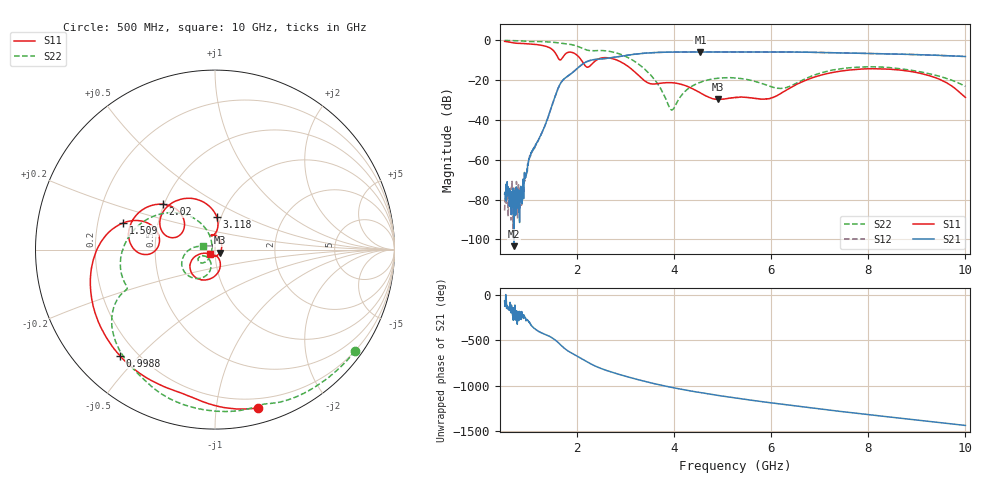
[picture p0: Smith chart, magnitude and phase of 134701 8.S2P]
!  2-Port S-parameters saved by WinCal
! VAR MeasName=S-Parameters (CALIBRATED_DATA) read from VNA (N5242A)
! VAR MeasDate=2013-7-3 16:23:51
! VAR NAME=134701 8
! VAR FILENAME=134701 8.S2P
! VAR DATE=2013-7-3 16:23:51
! VAR PHYS_PORTS=1,2
# Hz S MA R 50
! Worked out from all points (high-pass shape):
!   1601 points, 500 MHz to 10 GHz, reference 50 ohm
!   highest |S21| = -6.07 dB at 4.537 GHz (marker M1); lowest = -103.3 dB at 695.9 MHz (marker M2)
!   |S21| within 3 dB of the highest: 2.671 GHz to end of sweep
!   lowest |S11| = -29.8 dB at 4.9 GHz (marker M3), VSWR 1.07, Z = 52.8 - j1.8 ohm
!   |S11| at or under -10 dB: 1.633 GHz to 1.658 GHz (24.43 MHz wide, 1.49 % of centre); 2.077 GHz to 2.404 GHz (327.1 MHz wide, 14.6 % of centre); 2.799 GHz to end of sweep
!   |S22| runs from -35.2 to -0.3 dB; largest |S21 - S12| = 0.0018
!   S11 on the Smith chart (normalised r, x): 500 MHz: 0.12, -1.30; 998.8 MHz: 0.14, -0.44; 1.509 GHz: 0.31, +0.13; 2.02 GHz: 0.49, +0.29; 3.118 GHz: 0.95, +0.36; 10 GHz: 0.95, -0.05
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5e8  0.9137 -74.9  0.0001384 -68.9  5.323e-05 148.5  0.9632 -35.9
6.959375e8  0.8312 -99.3  6.8e-06 -173.9  0.0001253 135.1  0.9513 -49.8
8.503125e8  0.8112 -115.3  0.0001051 175.3  7.243e-05 95.9  0.9374 -60.9
9.9875e8  0.7937 -132.0  0.001044 65.2  0.0009223 63.8  0.9076 -71.1
1.289688e9  0.7167 -165.8  0.005374 -66.0  0.005442 -66.4  0.8986 -90.9
1.509375e9  0.5329 163.8  0.02984 -124.7  0.02959 -124.7  0.866 -107.7
1.681562e9  0.3405 -178.0  0.09147 155.2  0.09116 155.0  0.8176 -120.6
2.02e9  0.3841 138.9  0.2028 37.6  0.2021 37.6  0.6756 -148.0
2.085312e9  0.3059 133.6  0.2362 17.7  0.2353 17.7  0.6259 -152.0
2.221875e9  0.2067 153.7  0.2941 -24.3  0.2932 -24.4  0.5454 -155.6
2.51875e9  0.3542 147.8  0.3346 -97.1  0.3334 -97.1  0.5372 -168.1
3.118438e9  0.1837 87.2  0.4266 165.3  0.4261 165.4  0.3207 140.0
3.670625e9  0.07982 107.3  0.4839 92.1  0.4828 92.1  0.07391 111.0
3.949688e9  0.08444 99.1  0.4927 60.6  0.4924 60.7  0.01744 176.0
4.5375e9  0.04691 37.1  0.4973 3.6  0.4966 3.6  0.08681 -128.0
4.899688e9  0.03226 -31.9  0.4959 -27.2  0.4959 -27.2  0.1091 -137.9
5.25e9  0.03588 -83.1  0.4954 -54.8  0.4954 -54.8  0.1107 -148.1
6.2e9  0.04573 -70.1  0.4951 -123.0  0.4956 -123.1  0.06062 -129.7
6.835312e9  0.1106 -76.4  0.4865 -165.9  0.4867 -165.8  0.1245 -103.6
8.420625e9  0.1843 -135.1  0.4429 96.6  0.4419 96.5  0.2024 -156.7
9.376562e9  0.113 -161.7  0.411 39.8  0.4113 39.7  0.1301 176.7
1e10  0.03609 -136.8  0.3814 2.7  0.3812 2.7  0.06829 165.0
